(* Logix 5000 AddOnInstructionDefinition export; software revision 16.04 *)

TYPE ST_PARKER_PDInParser_P8S :   // This data structure includes the process data inputs of the IO-Link device
STRUCT
   Positionin1mm128 : P8S_Positionin1mm128;   // Positionin1mm128
END_STRUCT
END_TYPE

TYPE P8S_Positionin1mm128 :   // This data type includes the device values of the corresponding data structure
STRUCT
   NoName : INT;   // [Integer]
END_STRUCT
END_TYPE

ADD_ON_INSTRUCTION F_PARKER_PDInParser_P8S   (* revision 1.6, vendor Parker Hannifin GmbH *)
// PARKER FB_PARKER_P8S process data parser IO-Link AOI
// Revision note:
// Generator version: 1.9.0.1000R
// Help:
// This AOI interprets the incoming process data. The normalizes data are stored in the referenced structure ST_PARKER_PDInParser_P8S.
// Please note: Do not change the origin byte order of the raw process data
VAR_IN_OUT
   arrRawData : SINT[1]; {required}   // Raw input process data
   stProcessData : ST_PARKER_PDInParser_P8S; {required}   // Process data
END_VAR
VAR
   arrTempItem : SINT[232];   // Temporarily data
   arrIOLRecord : SINT[232];   // Temporarily data
   arrTemp : SINT[4];   // Temporarily variable
   iIndex : INT;   // Temporarily index variable
END_VAR

ROUTINE Logic   (* structured text *)
   (*=================================================================================
   Name: P8S IO-Link process data Add-On Instruction
   Company: Parker Hannifin GmbH
   Date: Wed Apr 25 10:59:19 CEST 2018
   Generator Version: V1.9.0.1000R
   IODD Version: V1.3
   -----------------------------------------------------------------------------------
   Description:
   This function helps you to interpret the incoming process data from the
   PARKER IO-Link device on Rockwell ControlLogix / CompactLogix PLCs.
   
   This AOI is only suitable with RSLogix5000 V16 or higher.
   =================================================================================*)
   (*Copy process data input*)
   COP(arrRawData[0], arrIOLRecord[0], 2);
   
   		(**)
   		COP(arrIOLRecord[0], arrTemp[0], 2);
   		arrTempItem[0]:= arrTemp[1];
   		arrTempItem[1]:= arrTemp[0];
   		COP(arrTempItem[0], stProcessData.Positionin1mm128.NoName, 1);
END_ROUTINE
END_ADD_ON_INSTRUCTION
